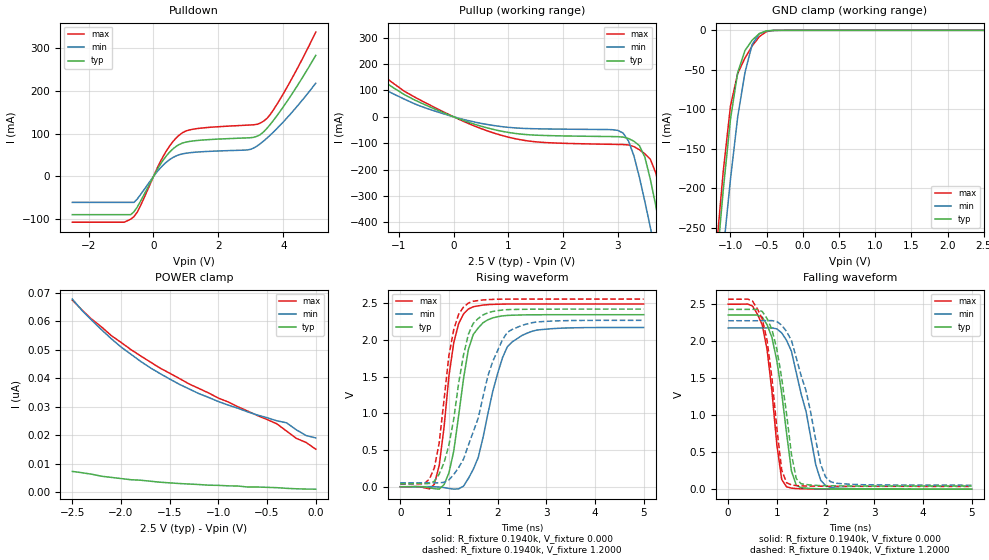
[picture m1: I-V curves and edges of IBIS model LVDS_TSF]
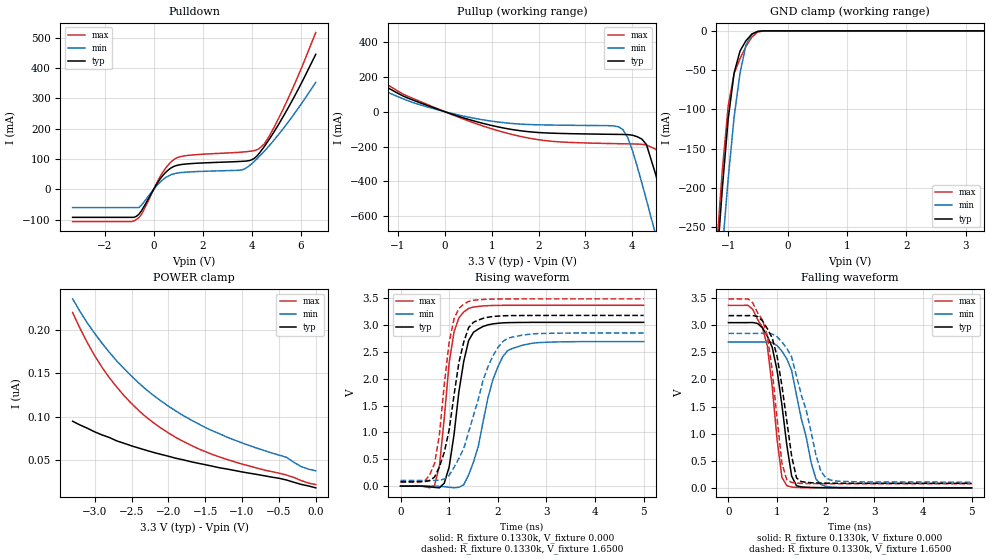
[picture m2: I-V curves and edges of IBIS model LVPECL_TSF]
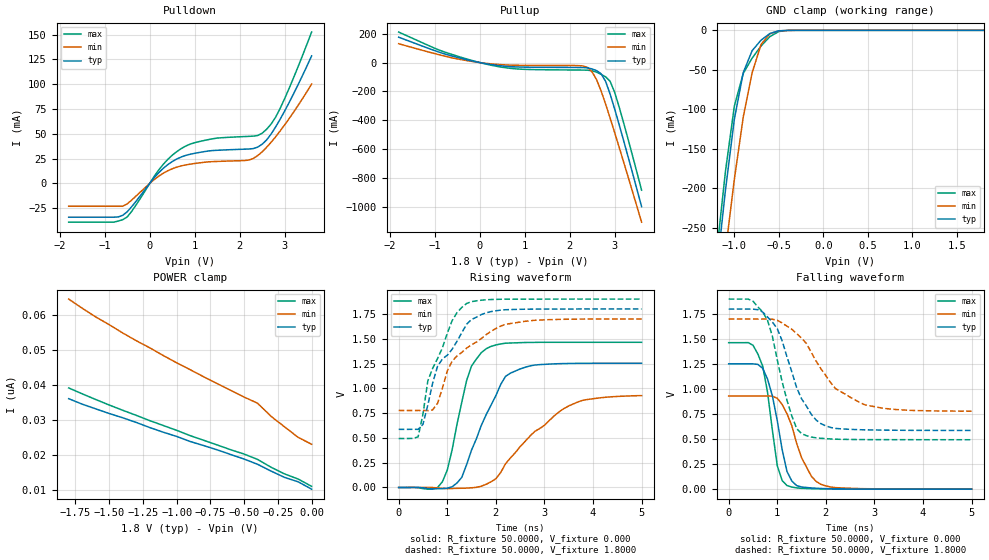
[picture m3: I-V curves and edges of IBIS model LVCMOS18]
| / 7\'7
| \ \   Xilinx Inc.
| / /
| \_\/.\   IBIS Models for Virtex-E
[IBIS ver]   2.1
[File name]   virtexe.ibs
[File Rev]   1.3
[Date]   Jun. 12, 2002
[Source]   Hspice simulations (18-07: TT, SS, FF, FS, SF)
[Notes]   Xilinx IBIS model for Virtex-E I/O.
   The package models are provided for BG432, BG560, BG728,
   HQ240, PQ240, CS144, FG256, FG456, FG676, FG680, FG860,
   FG900, and FG1156 package types,
   with BG432 being selected as a default. Please make your
   own selection of the packages by commenting out the
   unused ones.
   VirtexE LVDS and LVPECL drivers require the use of external
   resistors to provide the correct voltage levels.
   Please read Xilinx application note XAPP232 "Virtex-E LVDS
   (LVPECL) Drivers& Receivers:  Interface Guidelines" for details
   The values for Vref specified below refer to the IBIS
   Vref (the voltage to which the load resistor is connected in
   the IBIS model) and not the Vref of the corresponding
   differential input standard.
   These 2 Vrefs will not necessarily have the same value for a
   given standard.
   The HSTL models are based on 1.8V Vcco.
   COMMENTS: Models include process corners for MIN and MAX.
   See [Pin] section for details.
[Disclaimer] The data in this model is derived from SPICE simulations using
   modeling information extracted from the target process. While
   a great deal of care has been taken to provide information
   that is accurate, this model is considered preliminary as it
   has not been verified by actual silicon measurement. Treat the
   data in this model as preliminary until actual silicon
   verification is performed.
[Copyright]   Copyright 2002, Xilinx Inc., All rights reserved
|   Component Virtex-E
|   >>> Make Your Selection of the Package type Below <<<
[Component]   VIRTEX-E
[Manufacturer]   Xilinx Inc.
[Package]
| For Package type BG432:
| variable   typ   min   max
R_pkg   0.258   0.1870   0.3280
L_pkg   5.1nH   2.4000nH   7.8000nH
C_pkg   1.1pF   0.8000pF   1.4000pF
| For Package type BG352:
| variable   typ   min   max
|R_pkg   0.2340   0.1640   0.3040
|L_pkg   6.5500nH   3.8000nH   9.3000nH
|C_pkg   1.0200pF   0.7300pF   1.3100pF
| For Package type BG560:
| variable   typ   min   max
|R_pkg   0.265   0.1630   0.5510
|L_pkg   6.4nH   2.2000nH   10.700nH
|C_pkg   0.93pF   0.2600pF   2.6800pF
| For Package type BG728_XCV1000E:
| variable   typ   min   max
|R_pkg   179m   116m   276m
|L_pkg   5.3nH   2.8nH   10.3nH
|C_pkg   0.5pF   0.2pF   1.1pF
| For Package type HQ240:
| variable   typ   min   max
|R_pkg   0.180   0.163   0.198
|L_pkg   12.95nH   8.60nH   17.3nH
|C_pkg   2.2pF   1.90pF   2.50pF
| For Package type PQ240:
| variable   typ   min   max
|R_pkg   0.201   0.195   0.207
|L_pkg   18.85nH   11.9nH   25.8nH
|C_pkg   1.6pF   1.30pF   1.90pF
| For Package type CS144:
| variable   typ   min   max
|R_pkg   0.116   0.078   0.153
|L_pkg   3.55nH   1.5nH   5.60nH
|C_pkg   0.6pF   0.50pF   0.70pF
| For Package type FG256:
| variable   typ   min   max
|R_pkg   0.141   0.073   0.230
|L_pkg   4.06nH   1.69nH   6.80nH
|C_pkg   0.68pF   0.47pF   1.17pF
| For Package type FG456:
| variable   typ   min   max
|R_pkg   0.155   0.087   0.231
|L_pkg   4.42nH   1.8nH   7.40nH
|C_pkg   0.85pF   0.50pF   1.50pF
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[Pin]  signal_name   model_name   R_pin   L_pin   C_pin
1   LVDS_MIX+   LVDS_MIX
2   LVDS_MIX-   LVDS_MIX
3   LVDS_TSF+   LVDS_TSF
4   LVDS_TSF-   LVDS_TSF
5   LVPECL_MIX+   LVPECL_MIX
6   LVPECL_MIX-   LVPECL_MIX
7   LVPECL_TSF+   LVPECL_TSF
8   LVPECL_TSF-   LVPECL_TSF
9   LVCMOS18   LVCMOS18
10   LVCMOS25   LVCMOS25
11   LVTTL2F   LVTTL2F
12   LVTTL4F   LVTTL4F
13   LVTTL6F   LVTTL6F
14   LVTTL8F   LVTTL8F
15   LVTTL12F   LVTTL12F
16   LVTTL16F   LVTTL16F
17   LVTTL24F   LVTTL24F
18   LVTTL2S   LVTTL2S
19   LVTTL4S   LVTTL4S
20   LVTTL6S   LVTTL6S
21   LVTTL8S   LVTTL8S
22   LVTTL12S   LVTTL12S
23   LVTTL16S   LVTTL16S
24   LVTTL24S   LVTTL24S
25   HSTL1   HSTL1
26   HSTL3   HSTL3
27   HSTL4   HSTL4
28   SSTL21   SSTL21
29   SSTL22   SSTL22
30   SSTL31   SSTL31
31   SSTL32   SSTL32
32   CTT   CTT
33   AGP   AGP
34   GTL   GTL
35   GTL-PLUS   GTL-PLUS
36   PCI33M   PCI33M
37   PCI66M   PCI66M
PGND   GND   GND
VCCO   VCCO   POWER
[Diff Pin]   inv_pin   vdiff   tdelay_typ   tdelay_min   tdelay_max
| Here is just a sample format for differential pin pairs.
| Edit the list based on your applications.
1   2   300mV   0   0   0
3   4   300mV   0   0   0
5   6   300mV   0   0   0
7   8   300mV   0   0   0
| Models and submodels in the file (33): LVDS_TSF (I/O), LVDS_MIX (I/O), LVPECL_TSF (I/O), LVPECL_MIX (I/O), LVCMOS18 (I/O), LVCMOS25 (I/O), LVTTL2F (I/O), LVTTL4F (I/O), LVTTL6F (I/O), LVTTL8F (I/O), LVTTL12F (I/O), LVTTL16F (I/O), LVTTL24F (I/O), LVTTL2S (I/O), LVTTL4S (I/O), LVTTL6S (I/O), LVTTL8S (I/O), LVTTL12S (I/O), LVTTL16S (I/O), LVTTL24S (I/O), HSTL1 (I/O), HSTL3 (I/O), HSTL4 (I/O), SSTL21 (I/O), SSTL22 (I/O), SSTL31 (I/O), SSTL32 (I/O), CTT (I/O), AGP (I/O), GTL (I/O_open_drain), GTL-PLUS (I/O_open_drain), PCI33M (I/O), PCI66M (I/O)
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|   Model LVDS_TSF
[Model]   LVDS_TSF
Model_type   I/O
Polarity   Non-Inverting
Enable   Active-Low
Vinh  = 1.4V
Vinl  = 1.0V
Vmeas =   1.2000V
Cref =  10.0000pF
Rref =   1.0000M
Vref =  0.000V
C_comp   5.0000pF   4.0000pF   6.0000pF
[Temperature Range]   25.0000   100.0000   0.000
[Voltage Range]   2.5000V   2.3750V   2.6250V
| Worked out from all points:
|   slope of the pulldown table from 0 to 0.375 V, typ, clamps not added: 8.2 ohm
|   slope of the pullup table from 0 to 0.375 V, typ, clamps not added: 13.6 ohm
|   GND clamp passes 1 mA (typ) near -0.51 V on its own axis
|   rising waveform, R_fixture 0.1940k, V_fixture 0.000: 20-80 % time 308ps typ, 476ps min, 271ps max; typ from 0 V to 2.35 V
|   rising waveform, R_fixture 0.1940k, V_fixture 1.2000: 20-80 % time 374ps typ, 616ps min, 290ps max; typ from 0.041 V to 2.42 V
|   falling waveform, R_fixture 0.1940k, V_fixture 0.000: 20-80 % time 303ps typ, 429ps min, 256ps max; typ from 2.35 V to 0 V
|   falling waveform, R_fixture 0.1940k, V_fixture 1.2000: 20-80 % time 315ps typ, 474ps min, 267ps max; typ from 2.42 V to 0.041 V
[Pulldown]
| voltage   I(typ)   I(min)   I(max)
-2.5V     -88.86mA   -60.26mA   -106.4mA
-900mV    -88.86mA   -60.26mA   -106.4mA
-600mV    -82.12mA   -60.26mA   -93.33mA
-400mV    -57.77mA   -42.35mA   -68.09mA
300mV     38.21mA    26.69mA    46.99mA
600mV     64.23mA    44.18mA    81.23mA
900mV     77.98mA    52.75mA    102.2mA
2.9V      89.95mA    61.9mA     119.6mA
3.4V      104.3mA    82.96mA    129.3mA
3.6V      121.4mA    96.48mA    144.6mA
4V        162.1mA    127mA      192.5mA
5V        282mA      217.1mA    336.2mA
[Pullup]
| voltage   I(typ)   I(min)   I(max)
-2.5V     295.5mA    231.1mA    340.7mA
-900mV    83.9mA     66.74mA    96.64mA
400mV     -29.28mA   -20.55mA   -36.46mA
1.4V      -68.49mA   -44.87mA   -92.63mA
3V        -75.36mA   -51.4mA    -104.8mA
3.2V      -82.3mA    -91.8mA    -106.8mA
3.3V      -92.74mA   -149mA     -113.1mA
3.5V      -153.5mA   -322.4mA   -140.6mA
3.6V      -237.5mA   -419.7mA   -161mA
3.8V      -446.3mA   -621.6mA   -305.8mA
4V        -670.1mA   -828.4mA   -525.3mA
5V        -1.834A    -1.888A    -1.72A
[GND_clamp]
| voltage   I(typ)   I(min)   I(max)
-2.5V     -1.803A    -1.736A    -1.828A
-1.2V     -306mA     -377.1mA   -282.8mA
-1.1V     -202.6mA   -280mA     -178.8mA
-1V       -112.6mA   -188.5mA   -96.01mA
-900mV    -53.5mA    -109.7mA   -54.54mA
-800mV    -25.67mA   -53.6mA    -35.14mA
-700mV    -12.44mA   -17.88mA   -19.83mA
-600mV    -3.983mA   -4.202mA   -7.871mA
-500mV    -601.8uA   -800.4uA   -1.51mA
-400mV    -51.06uA   -119.3uA   -124.5uA
2.5V      1.193nA    51.4nA     1.659nA
[POWER_clamp]
| voltage   I(typ)   I(min)   I(max)
-2.5V     7.392nA    67.87nA    67.52nA
-2.3V     6.403nA    60.42nA    60.77nA
-2V       4.889nA    51.05nA    52.68nA
-1.8V     4.307nA    46.04nA    47.96nA
-1.6V     3.609nA    41.73nA    43.66nA
-1.4V     3.143nA    37.95nA    39.99nA
-1V       2.503nA    31.9nA     33.12nA
-400mV    1.688nA    25.15nA    24.1nA
-300mV    1.455nA    24.45nA    21.54nA
-200mV    1.3nA      22nA       19nA
-100mV    1.2nA      20nA       17.58nA
0V        1.164nA    19.15nA    15.19nA
[Ramp]
| variable   typ   min   max
dV/dt_r   1.4070/0.3280n   1.3026/0.4908n   1.4946/0.2610n
dV/dt_f   1.4472/0.3288n   1.3535/0.4905n   1.5291/0.2665n
R_load = 0.1940k
[Rising Waveform]
R_fixture = 0.1940k
V_fixture = 0.000
| time   V(typ)   V(min)   V(max)
0s        24.75uV    13.64uV    77.86uV
700ps     -26.98mV   239.6uV    32.66mV
800ps     -32.13mV   -4.577mV   289.2mV
1ns       187.7mV    -22.82mV   1.51V
1.2ns     971.1mV    -28.25mV   2.224V
1.4ns     1.872V     113.7mV    2.422V
1.7ns     2.235V     669.4mV    2.476V
2ns       2.317V     1.542V     2.487V
2.3ns     2.338V     1.974V     2.491V
5ns       2.345V     2.171V     2.491V
[Rising Waveform]
R_fixture = 0.1940k
V_fixture = 1.2000
V_fixture_min = 1.1000
V_fixture_max = 1.3000
| time   V(typ)   V(min)   V(max)
0s        41.3mV     53.11mV    37.33mV
600ps     44.23mV    54.78mV    106.4mV
800ps     172.4mV    53.3mV     595.9mV
1ns       568.2mV    92.06mV    1.79V
1.1ns     927.4mV    167.2mV    2.144V
1.4ns     2.079V     566.9mV    2.504V
1.9ns     2.389V     1.707V     2.554V
2.2ns     2.414V     2.104V     2.557V
2.8ns     2.42V      2.245V     2.558V
5ns       2.421V     2.268V     2.558V
[Falling Waveform]
R_fixture = 0.1940k
V_fixture = 0.000
| time   V(typ)   V(min)   V(max)
0s        2.345V     2.171V     2.491V
700ps     2.316V     2.171V     2.213V
800ps     2.213V     2.172V     1.878V
1ns       1.73V      2.159V     597.4mV
1.1ns     1.29V      2.104V     131mV
1.2ns     752.5mV    2.004V     32.2mV
1.4ns     51.59mV    1.566V     8.174mV
1.8ns     6.647mV    327.1mV    2.475mV
2ns       3.765mV    48.82mV    1.564mV
5ns       206.7uV    455.5uV    236.7uV
[Falling Waveform]
R_fixture = 0.1940k
V_fixture = 1.2000
V_fixture_min = 1.1000
V_fixture_max = 1.3000
| time   V(typ)   V(min)   V(max)
0s        2.421V     2.268V     2.558V
700ps     2.393V     2.268V     2.296V
800ps     2.297V     2.269V     2.002V
1ns       1.885V     2.257V     822.7mV
1.1ns     1.494V     2.208V     254.8mV
1.2ns     1.013V     2.123V     86.57mV
1.4ns     140.8mV    1.768V     48.33mV
1.9ns     48.62mV    335.6mV    39.72mV
2.1ns     45.33mV    102.3mV    38.73mV
5ns       41.48mV    53.63mV    37.52mV
|   Model LVPECL_TSF
[Model]   LVPECL_TSF
Model_type   I/O
Polarity   Non-Inverting
Enable   Active-Low
Vinh  = 1.49V
Vinl  = 0.86V
Vmeas =   1.6500V
Cref =  10.0000pF
Rref =   1.0000M
Vref =  0.000V
C_comp   5.0000pF   4.0000pF   6.0000pF
[Temperature Range]   25.0000   100.0000   0.000
[Voltage Range]   3.3000V   3.0000V   3.6000V
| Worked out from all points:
|   slope of the pulldown table from 0 to 0.495 V, typ, clamps not added: 8.76 ohm
|   slope of the pullup table from 0 to 0.495 V, typ, clamps not added: 11.4 ohm
|   GND clamp passes 1 mA (typ) near -0.51 V on its own axis
|   rising waveform, R_fixture 0.1330k, V_fixture 0.000: 20-80 % time 288ps typ, 443ps min, 236ps max; typ from 0 V to 3.05 V
|   rising waveform, R_fixture 0.1330k, V_fixture 1.6500: 20-80 % time 351ps typ, 563ps min, 267ps max; typ from 0.083 V to 3.18 V
|   falling waveform, R_fixture 0.1330k, V_fixture 0.000: 20-80 % time 295ps typ, 382ps min, 255ps max; typ from 3.05 V to 0 V
|   falling waveform, R_fixture 0.1330k, V_fixture 1.6500: 20-80 % time 321ps typ, 456ps min, 263ps max; typ from 3.18 V to 0.083 V
[Pulldown]
| voltage   I(typ)   I(min)   I(max)
-3.3V     -92.53mA   -60.26mA   -106.4mA
-800mV    -92.53mA   -60.26mA   -104.2mA
-500mV    -71.29mA   -52.47mA   -83.03mA
400mV     48.26mA    33.54mA    59.86mA
900mV     78mA       52.76mA    102.3mA
3.6V      92.45mA    64.36mA    123mA
4V        97.87mA    85.07mA    126.6mA
4.3V      119mA      108.2mA    134.8mA
4.7V      164.4mA    143.4mA    174.7mA
5.1V      216.1mA    182.4mA    236.1mA
5.9V      332.5mA    269.2mA    377.9mA
6.6V      445.8mA    353.1mA    517.5mA
[Pullup]
| voltage   I(typ)   I(min)   I(max)
-3.3V     429mA      345mA      481.4mA
-900mV    91.79mA    75.42mA    102.6mA
600mV     -51.47mA   -36.4mA    -62.21mA
2V        -119.7mA   -75.41mA   -160.9mA
3.7V      -130.4mA   -86.33mA   -183.7mA
3.9V      -131.6mA   -148.1mA   -184.7mA
4.2V      -156.7mA   -407.1mA   -186.8mA
4.5V      -362.9mA   -710mA     -215.9mA
4.7V      -579.5mA   -917.8mA   -285.2mA
4.9V      -805.7mA   -1.127A    -476.4mA
5.1V      -1.036A    -1.339A    -703.2mA
6.6V      -2.802A    -2.947A    -2.515A
[GND_clamp]
| voltage   I(typ)   I(min)   I(max)
-3.3V     -2.749A    -2.594A    -2.805A
-1.2V     -306mA     -377mA     -282.7mA
-1.1V     -202.5mA   -280mA     -178.8mA
-1V       -112.5mA   -188.5mA   -95.98mA
-900mV    -53.5mA    -109.7mA   -54.53mA
-800mV    -25.67mA   -53.59mA   -35.13mA
-700mV    -12.44mA   -17.88mA   -19.82mA
-600mV    -3.982mA   -4.202mA   -7.865mA
-500mV    -601.5uA   -800.4uA   -1.508mA
-400mV    -51.05uA   -119.4uA   -124.3uA
3.3V      18.51nA    1.016uA    17.81nA
[POWER_clamp]
| voltage   I(typ)   I(min)   I(max)
-3.3V     94.99nA    235.5nA    219.8nA
-3.1V     86.96nA    207.8nA    185.2nA
-2.8V     76.25nA    174nA      144.8nA
-2.5V     66.71nA    146.8nA    115.3nA
-2.3V     61.58nA    131.3nA    99.65nA
-2.1V     56.93nA    118.3nA    87.08nA
-1.8V     50.7nA     101.6nA    71.94nA
-1.4V     43.31nA    83.94nA    56.75nA
-1V       36.79nA    70.08nA    45.81nA
-400mV    27.59nA    53.67nA    33.24nA
-200mV    22.5nA     43nA       27nA
0V        18.51nA    38.07nA    22.24nA
[Ramp]
| variable   typ   min   max
dV/dt_r   1.8282/0.2770n   1.6140/0.4212n   2.0190/0.2208n
dV/dt_f   1.8761/0.3456n   1.6648/0.5143n   2.0666/0.2768n
R_load = 0.1330k
[Rising Waveform]
R_fixture = 0.1330k
V_fixture = 0.000
| time   V(typ)   V(min)   V(max)
0s        1.448uV    1.712uV    1.4uV
700ps     -23.45mV   535.8uV    15.39mV
800ps     -31.34mV   -3.63mV    373.3mV
1ns       355.8mV    -20.14mV   2.293V
1.1ns     956.7mV    -30.53mV   2.866V
1.3ns     2.321V     26.28mV    3.24V
1.5ns     2.863V     448.6mV    3.332V
1.9ns     3.019V     1.982V     3.361V
2.2ns     3.042V     2.519V     3.365V
5ns       3.047V     2.69V      3.365V
[Rising Waveform]
R_fixture = 0.1330k
V_fixture = 1.6500
V_fixture_min = 1.5000
V_fixture_max = 1.8000
| time   V(typ)   V(min)   V(max)
0s        83.01mV    106mV      75.33mV
500ps     86.4mV     106.9mV    98.23mV
700ps     170.9mV    107.2mV    423.6mV
800ps     359.6mV    110.8mV    958.7mV
1ns       1.048V     202mV      2.676V
1.1ns     1.692V     349.5mV    3.112V
1.3ns     2.681V     700.2mV    3.386V
1.8ns     3.143V     2.226V     3.478V
2.2ns     3.171V     2.748V     3.483V
5ns       3.176V     2.849V     3.484V
[Falling Waveform]
R_fixture = 0.1330k
V_fixture = 0.000
| time   V(typ)   V(min)   V(max)
0s        3.047V     2.69V      3.365V
700ps     2.95V      2.69V      2.961V
800ps     2.796V     2.691V     2.611V
1ns       2.167V     2.624V     894.3mV
1.1ns     1.526V     2.519V     192.7mV
1.2ns     789.9mV    2.38V      40.25mV
1.4ns     38.89mV    1.705V     7.459mV
1.7ns     7.263mV    466.8mV    2.841mV
1.9ns     3.841mV    61.16mV    1.706mV
5ns       164.1uV    401uV      107.9uV
[Falling Waveform]
R_fixture = 0.1330k
V_fixture = 1.6500
V_fixture_min = 1.5000
V_fixture_max = 1.8000
| time   V(typ)   V(min)   V(max)
0s        3.176V     2.849V     3.484V
400ps     3.176V     2.849V     3.485V
700ps     3.079V     2.85V      3.096V
800ps     2.936V     2.85V      2.807V
1ns       2.426V     2.785V     1.278V
1.1ns     1.881V     2.691V     454.9mV
1.2ns     1.234V     2.575V     149.5mV
1.4ns     182.3mV    2.059V     86.07mV
2ns       86.88mV    186.4mV    76.91mV
5ns       83.25mV    106.4mV    75.43mV
|   Model LVCMOS18
[Model]   LVCMOS18
Model_type   I/O
Polarity   Non-Inverting
Enable   Active-Low
Vinh  = 1.26V
Vinl  = 0.36V
Vmeas =   0.9000V
Cref =  35.0000pF
Rref =   1.0000M
Vref =  0.000V
C_comp   5.0000pF   4.0000pF   6.0000pF
[Temperature Range]   25.0000   100.0000   0.000
[Voltage Range]   1.8000V   1.7000V   1.9000V
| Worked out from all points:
|   slope of the pulldown table from 0 to 0.27 V, typ, clamps not added: 19.5 ohm
|   slope of the pullup table from 0 to 0.27 V, typ, clamps not added: 18.5 ohm
|   GND clamp passes 1 mA (typ) near -0.51 V on its own axis
|   rising waveform, R_fixture 50.0000, V_fixture 0.000: 20-80 % time 655ps typ, 1.11ns min, 405ps max; typ from 0 V to 1.25 V
|   rising waveform, R_fixture 50.0000, V_fixture 1.8000: 20-80 % time 696ps typ, 858ps min, 540ps max; typ from 0.586 V to 1.8 V
|   falling waveform, R_fixture 50.0000, V_fixture 0.000: 20-80 % time 308ps typ, 432ps min, 261ps max; typ from 1.25 V to 0 V
|   falling waveform, R_fixture 50.0000, V_fixture 1.8000: 20-80 % time 562ps typ, 861ps min, 430ps max; typ from 1.8 V to 0.587 V
[Pulldown]
| voltage   I(typ)   I(min)   I(max)
-1.8V     -33.98mA   -22.94mA   -39mA
-800mV    -33.98mA   -22.94mA   -39mA
-600mV    -32.1mA    -22.94mA   -36.54mA
-400mV    -23.39mA   -16.72mA   -28.16mA
200mV     10.76mA    7.293mA    13.51mA
700mV     26.64mA    17.7mA     35.08mA
1.4V      33.18mA    22.01mA    45.01mA
2.2V      34.71mA    23.55mA    47.45mA
2.5V      39.51mA    31.91mA    50.58mA
2.7V      49.83mA    41.53mA    59.88mA
2.9V      64.67mA    52.83mA    75.57mA
3.6V      128.5mA    100.1mA    152.5mA
[Pullup]
| voltage   I(typ)   I(min)   I(max)
-1.8V     175.7mA    130.6mA    211.2mA
-800mV    61.82mA    46.12mA    75.32mA
300mV     -16.04mA   -10.52mA   -21.5mA
900mV     -31.21mA   -19.23mA   -45.78mA
2.4V      -37.11mA   -34.21mA   -52.96mA
2.6V      -56.17mA   -119.2mA   -67.3mA
2.7V      -77.8mA    -197.1mA   -81.73mA
2.8V      -130.7mA   -288.2mA   -99.11mA
2.9V      -218.5mA   -385mA     -130.1mA
3V        -321.2mA   -484.8mA   -205.6mA
3.1V      -429.6mA   -586.4mA   -307.2mA
3.6V      -999.2mA   -1.107A    -885mA
[GND_clamp]
| voltage   I(typ)   I(min)   I(max)
-1.8V     -984.4mA   -994.3mA   -981.6mA
-1.2V     -306mA     -377mA     -282.7mA
-1.1V     -202.5mA   -280mA     -178.7mA
-1V       -112.5mA   -188.5mA   -95.97mA
-900mV    -53.49mA   -109.7mA   -54.52mA
-800mV    -25.66mA   -53.59mA   -35.12mA
-700mV    -12.43mA   -17.88mA   -19.81mA
-600mV    -3.981mA   -4.201mA   -7.864mA
-500mV    -601.5uA   -800.2uA   -1.508mA
-400mV    -51.04uA   -119.3uA   -124.3uA
1.8V      10.13nA    42.38nA    9.692nA
[POWER_clamp]
| voltage   I(typ)   I(min)   I(max)
-1.8V     36.09nA    64.67nA    39.17nA
-1.6V     33.18nA    59.55nA    35.86nA
-1.3V     29.28nA    52.74nA    31.32nA
-900mV    23.81nA    44.41nA    25.49nA
-800mV    22.64nA    42.38nA    24.16nA
-500mV    18.77nA    36.55nA    20.2nA
-400mV    17.26nA    34.78nA    18.66nA
-300mV    15.31nA    31nA       16.41nA
-200mV    13.5nA     28nA       14.5nA
-100mV    12.25nA    25nA       13.04nA
0V        10.13nA    23.02nA    10.94nA
[Ramp]
| variable   typ   min   max
dV/dt_r   0.7518/0.6396n   0.5558/1.0671n   0.8784/0.4210n
dV/dt_f   0.7277/0.5540n   0.5523/0.8467n   0.8435/0.4164n
R_load = 50.0000
[Rising Waveform]
R_fixture = 50.0000
V_fixture = 0.000
| time   V(typ)   V(min)   V(max)
0s        0V         0V         1.305uV
900ps     -11.2mV    -8.457mV   57.58mV
1ns       -7.19mV    -11.67mV   174.8mV
1.2ns     44.91mV    -8.349mV   636.7mV
1.4ns     232.6mV    -6.097mV   1.082V
1.8ns     733.7mV    32.24mV    1.399V
2.2ns     1.121V     239.6mV    1.455V
2.5ns     1.196V     412.3mV    1.46V
3.7ns     1.252V     864.6mV    1.464V
5ns       1.253V     926.3mV    1.464V
[Rising Waveform]
R_fixture = 50.0000
V_fixture = 1.8000
V_fixture_min = 1.7000
V_fixture_max = 1.9000
| time   V(typ)   V(min)   V(max)
0s        586.3mV    776.5mV    493.7mV
400ps     586.3mV    776.8mV    510.3mV
500ps     636.4mV    776.6mV    739.3mV
600ps     831.6mV    775mV      1.075V
800ps     1.222V     848.3mV    1.3V
1.1ns     1.394V     1.275V     1.683V
1.4ns     1.647V     1.406V     1.856V
1.7ns     1.744V     1.502V     1.889V
2.2ns     1.792V     1.645V     1.899V
5ns       1.8V       1.699V     1.9V
[Falling Waveform]
R_fixture = 50.0000
V_fixture = 0.000
| time   V(typ)   V(min)   V(max)
0s        1.253V     931mV      1.464V
400ps     1.253V     931mV      1.465V
600ps     1.247V     931mV      1.352V
700ps     1.208V     931.1mV    1.23V
800ps     1.101V     931.5mV    968.8mV
1ns       685.7mV    908.6mV    235.2mV
1.2ns     177.6mV    754.2mV    36.49mV
1.5ns     22.16mV    315.4mV    8.998mV
1.9ns     7.21mV     48.31mV    3.274mV
5ns       400.1uV    831.9uV    282.7uV
[Falling Waveform]
R_fixture = 50.0000
V_fixture = 1.8000
V_fixture_min = 1.7000
V_fixture_max = 1.9000
| time   V(typ)   V(min)   V(max)
0s        1.8V       1.7V       1.9V
500ps     1.799V     1.7V       1.879V
800ps     1.72V      1.7V       1.688V
1ns       1.605V     1.688V     1.292V
1.2ns     1.323V     1.629V     889mV
1.5ns     903.3mV    1.51V      555.1mV
1.9ns     654.7mV    1.202V     508.6mV
2.2ns     607.3mV    1.006V     499.6mV
2.8ns     593.2mV    844mV      495.6mV
5ns       587.2mV    779.5mV    494.2mV
